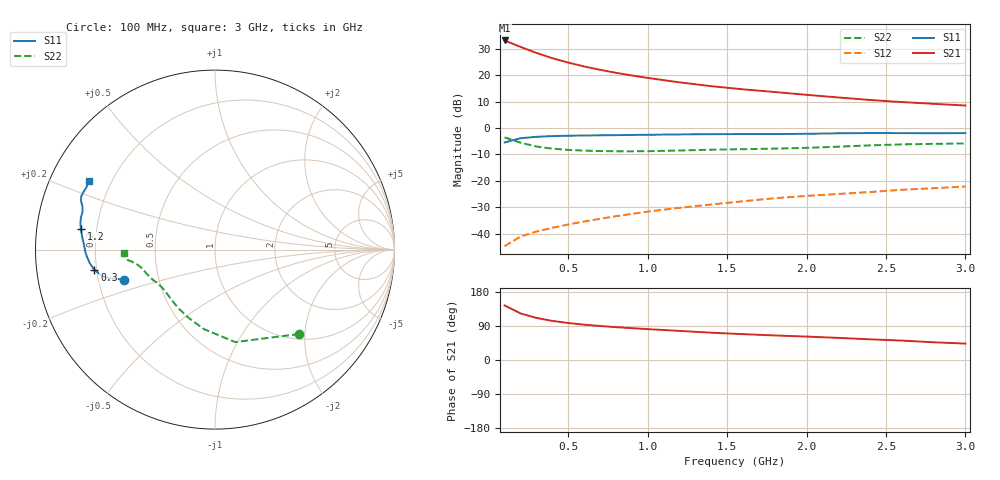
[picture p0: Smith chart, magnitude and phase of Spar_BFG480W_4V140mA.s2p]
! Filename: 4140BFG480.001
! Title: BFG480W
! Bias: Vce=4V; Ic=140mA
! Company: NXP Semiconductors NL
! User: Quality&Reliability T&D
! Measure time: 10 Nov 1999 / 12:04:49
#  MHz  S  MA  R 50
! Freq  S11  S21  S12  S22  :
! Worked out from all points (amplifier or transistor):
!   20 points, 100 MHz to 3 GHz, reference 50 ohm
!   highest |S21| = 33.2 dB at 100 MHz (marker M1)
!   |S21| within 3 dB of that: start of sweep to 224.7 MHz
!   unconditionally stable (mu >= 1): 509.9 MHz to end of sweep
!   at 400 MHz: K = 0.93, MSG = 32.1 dB, |S12| = -37.8 dB
!   at 1.2 GHz: K = 1.12, MAG = 21.7 dB, |S12| = -30.2 dB
!   at 3 GHz: K = 1.07, MAG = 13.7 dB, |S12| = -22.2 dB
!   S11 on the Smith chart (normalised r, x): 100 MHz: 0.31, -0.15; 300 MHz: 0.19, -0.08; 1.2 GHz: 0.14, +0.07; 3 GHz: 0.12, +0.25
100  0.5332 -161.6  45.5 143.9  0.005782 66.5  0.6641 -45.1
200  0.639 -166.1  34.38 122.9  0.008814 60.5  0.5275 -77.7
300  0.6812 -170.5  26.42 111.1  0.01092 60.9  0.4465 -98.2
400  0.7022 -173.9  21 103.2  0.01289 63.3  0.4062 -111.9
500  0.7131 -176.5  17.34 97.6  0.01488 65.9  0.3854 -121.5
600  0.7218 -178.7  14.65 93.3  0.01694 67.9  0.3735 -128.5
700  0.7268 179.3  12.67 89.7  0.01905 70.1  0.3663 -133.9
800  0.7319 177.4  11.12 86.7  0.02134 71.6  0.3625 -138.3
900  0.7388 175.7  9.876 84.0  0.02362 73.3  0.3616 -142.1
1000  0.745 174.1  8.884 81.5  0.02609 74.3  0.3639 -145.6
1200  0.7557 171.3  7.325 76.8  0.03076 75.6  0.375 -151.1
1400  0.7637 169.1  6.198 72.1  0.03555 76.5  0.3882 -155.1
1600  0.7681 166.8  5.404 68.2  0.04099 77.0  0.3972 -158.3
1800  0.7672 164.2  4.801 64.8  0.04681 77.3  0.4072 -161.8
2000  0.7761 162.1  4.249 61.8  0.05175 77.8  0.4212 -165.9
2200  0.794 160.1  3.791 58.3  0.05632 77.6  0.4427 -169.4
2400  0.8025 158.3  3.393 54.6  0.06128 76.9  0.4685 -171.8
2600  0.8002 156.6  3.098 51.2  0.06761 76.1  0.4895 -173.2
2800  0.7958 154.2  2.871 46.8  0.07239 74.7  0.5008 -175.0
3000  0.8008 151.6  2.665 43.3  0.0779 73.7  0.51 -177.8
